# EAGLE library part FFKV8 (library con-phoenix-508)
PHOENIX
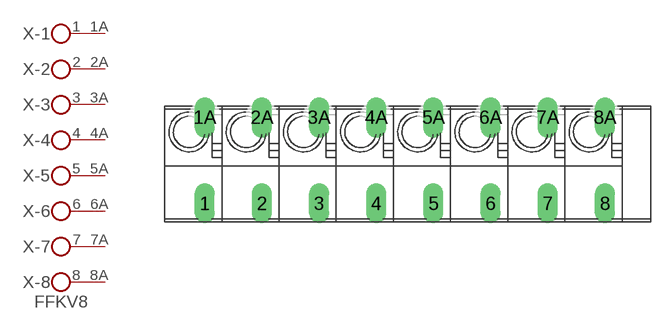
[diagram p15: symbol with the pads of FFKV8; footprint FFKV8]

Designator prefix X; gates -1=KL2 -2=KL2 -3=KL2 -4=KL2 -5=KL2 -6=KL2 -7=KL2 -8=KL2V

## FFKV8 (OC_FARNELL: unknown; OC_NEWARK: unknown)  [FFKV8]
1  -1:1  pas
1A  -1:2  pas
2  -2:1  pas
2A  -2:2  pas
3  -3:1  pas
3A  -3:2  pas
4  -4:1  pas
4A  -4:2  pas
5  -5:1  pas
5A  -5:2  pas
6  -6:1  pas
6A  -6:2  pas
7  -7:1  pas
7A  -7:2  pas
8  -8:1  pas
8A  -8:2  pas

## Footprint FFKV8 (pad centres in mm)
PHOENIX
drill 1.194 long: 1 -17.78,-3.81; 1A -17.78,3.81; 2 -12.7,-3.81; 2A -12.7,3.81; 3 -7.62,-3.81; 3A -7.62,3.81; 4 -2.54,-3.81; 4A -2.54,3.81; 5 2.54,-3.81; 5A 2.54,3.81; 6 7.62,-3.81; 6A 7.62,3.81; 7 12.7,-3.81; 7A 12.7,3.81; 8 17.78,-3.81; 8A 17.78,3.81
